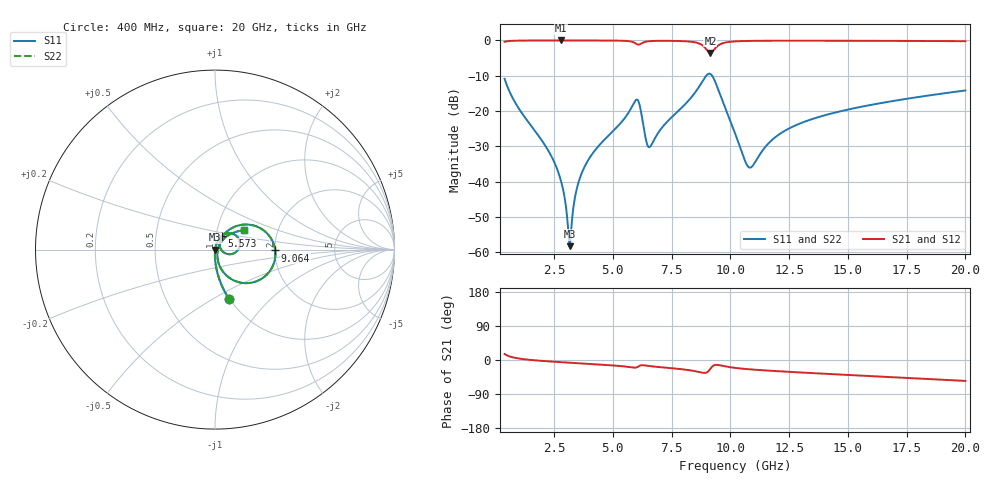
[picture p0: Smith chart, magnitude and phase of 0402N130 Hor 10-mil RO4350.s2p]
# GHz S MA R 50
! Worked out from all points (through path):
!   1960 points, 400 MHz to 20 GHz, reference 50 ohm
!   highest |S21| = -0.01 dB at 2.811 GHz (marker M1); lowest = -3.5 dB at 9.154 GHz (marker M2)
!   group delay of S21, straight-line fit = 7.9 ps
!   lowest |S11| = -58.3 dB at 3.171 GHz (marker M3), VSWR 1.00, Z = 50.1 - j0.00656 ohm
!   |S11| at or under -10 dB: start of sweep to 8.975 GHz; 9.228 GHz to end of sweep
!   |S22| runs from -58.3 to -9.4 dB; largest |S21 - S12| = 0
!   S11 on the Smith chart (normalised r, x): 400 MHz: 0.99, -0.59; 5.573 GHz: 1.06, +0.16; 9.064 GHz: 2.01, -0.02; 20 GHz: 1.35, +0.30
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0.4  0.2858 -74.2  0.9577 15.7  0.9577 15.7  0.2858 -74.2
1.020316  0.1066 -85.8  0.9935 3.8  0.9935 3.8  0.1066 -85.8
2.310975  0.02566 -91.5  0.9986 -3.8  0.9986 -3.8  0.02566 -91.5
2.81123  0.009887 -89.3  0.9987 -5.8  0.9987 -5.8  0.009887 -89.3
3.171414  0.001223 -3.1  0.9986 -7.2  0.9986 -7.2  0.001223 -3.1
3.421542  0.006717 70.7  0.9985 -8.2  0.9985 -8.2  0.006717 70.7
3.671669  0.01302 74.7  0.9984 -9.1  0.9984 -9.1  0.01302 74.7
4.22195  0.02719 75.1  0.9977 -11.2  0.9977 -11.2  0.02719 75.1
5.572639  0.08491 63.8  0.9834 -17.5  0.9834 -17.5  0.08491 63.8
6.032874  0.1452 20.1  0.8828 -19.0  0.8828 -19.0  0.1452 20.1
6.503114  0.03151 10.0  0.9712 -15.5  0.9712 -15.5  0.03151 10.0
6.943338  0.04977 57.1  0.9862 -18.5  0.9862 -18.5  0.04977 57.1
8.694232  0.2271 38.0  0.8988 -32.0  0.8988 -32.0  0.2271 38.0
9.064421  0.3356 -0.8  0.6929 -29.9  0.6929 -29.9  0.3356 -0.8
9.154467  0.3349 -15.8  0.6666 -23.2  0.6666 -23.2  0.3349 -15.8
9.594691  0.1611 -65.5  0.8905 -14.5  0.8905 -14.5  0.1611 -65.5
10.205  0.04812 -73.2  0.9695 -20.8  0.9695 -20.8  0.04812 -73.2
10.85533  0.01585 -7.6  0.9844 -24.7  0.9844 -24.7  0.01585 -7.6
11.92588  0.04297 49.0  0.9898 -29.2  0.9898 -29.2  0.04297 49.0
13.46667  0.07675 50.9  0.9903 -34.5  0.9903 -34.5  0.07675 50.9
16.73834  0.1356 43.0  0.9852 -44.9  0.9852 -44.9  0.1356 43.0
20  0.1957 33.5  0.9752 -55.2  0.9752 -55.2  0.1957 33.5
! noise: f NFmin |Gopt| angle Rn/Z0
0.4  0.001212  0.7783  1.453  0.001119
2.571  0.004363  0.6358  5.962  0.00225
4.752  0.009248  0.6757  10.62  0.005457
6.933  0.02403  0.8049  15.66  0.02511
9.104  0.1667  0.9601  20.57  0.9139
11.29  0.02937  0.7516  25.34  0.02273
13.47  0.02359  0.6549  29.73  0.0122
15.64  0.02315  0.6079  33.93  0.01005
17.82  0.02394  0.5809  38.01  0.009372
20  0.02522  0.5645  41.94  0.0092
